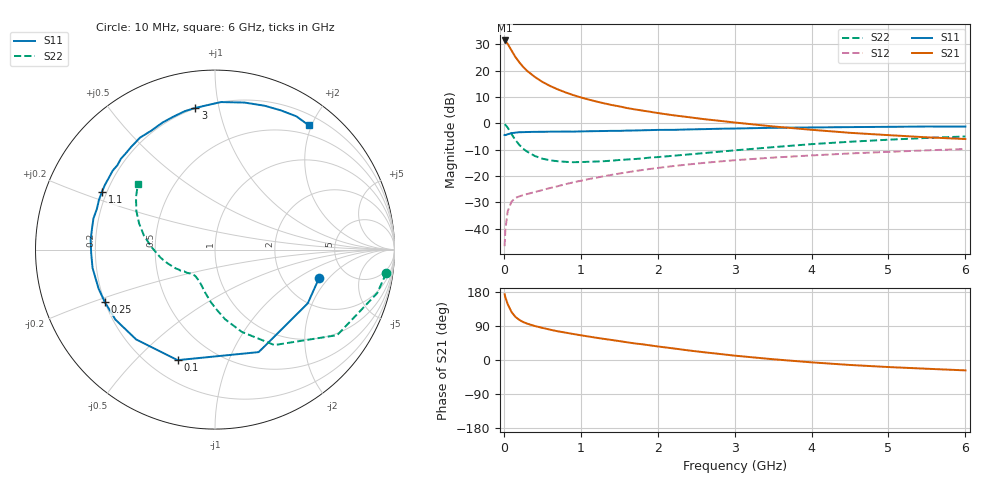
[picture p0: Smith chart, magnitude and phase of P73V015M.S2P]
! SIEMENS Small Signal Semiconductors
! BFP196
! Si NPN RF Bipolar Junction Transistor in SOT143
! VCE = 3 V  IC = 15 mA
! Common Emitter S-Parameters:  May  1996
# GHz  S  MA  R  50
!  f  S11  S21  S12  S22
! GHz  MAG  ANG  MAG  ANG  MAG  ANG  MAG  ANG
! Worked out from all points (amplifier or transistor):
!   36 points, 10 MHz to 6 GHz, reference 50 ohm
!   highest |S21| = 31.4 dB at 10 MHz (marker M1)
!   |S21| within 3 dB of that: start of sweep to 83.98 MHz
!   unconditionally stable (mu >= 1): 757.5 MHz to 3.338 GHz
!   at 250 MHz: K = 0.51, MSG = 24.3 dB, |S12| = -27.2 dB
!   at 1.4 GHz: K = 1.12, MAG = 11.1 dB, |S12| = -19.5 dB
!   at 6 GHz: K = 0.98, MSG = 1.9 dB, |S12| = -9.7 dB
!   S11 on the Smith chart (normalised r, x): 10 MHz: 3.18, -1.57; 100 MHz: 0.31, -0.67; 250 MHz: 0.20, -0.22; 1.1 GHz: 0.18, +0.23; 3 GHz: 0.20, +0.85; 6 GHz: 0.35, +1.96
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0.01  0.6013 -15.2  37.18 173.5  0.0047 84.9  0.9629 -7.8
0.02  0.5973 -30.1  35.97 165.5  0.0096 77.1  0.9358 -15.0
0.05  0.6208 -66.9  32.04 147.5  0.0215 62.9  0.8311 -35.0
0.1  0.6503 -108.7  23.99 126.6  0.0329 48.0  0.6264 -58.1
0.15  0.6661 -131.3  18.11 113.9  0.0385 40.7  0.4827 -71.9
0.2  0.6782 -144.9  14.4 106.0  0.0412 37.9  0.3927 -81.7
0.25  0.6799 -154.6  11.74 100.3  0.0436 37.0  0.3311 -88.9
0.3  0.6841 -161.4  9.954 96.2  0.0456 37.7  0.2932 -94.6
0.4  0.6899 -171.5  7.616 89.9  0.0497 39.2  0.2416 -103.8
0.5  0.6904 -178.7  6.109 84.8  0.0544 41.7  0.2138 -110.4
0.6  0.6949 175.4  5.116 80.1  0.0593 43.8  0.1993 -115.4
0.7  0.6952 170.2  4.406 75.8  0.0643 45.4  0.1911 -119.9
0.9  0.696 161.1  3.436 68.7  0.076 47.8  0.1835 -127.0
1.1  0.7075 152.9  2.827 62.0  0.0876 48.7  0.1867 -131.8
1.3  0.7145 145.5  2.399 55.7  0.0995 48.9  0.1916 -136.2
1.6  0.7287 136.0  1.949 46.8  0.1179 48.0  0.2063 -142.5
2.2  0.7517 118.2  1.423 30.7  0.1548 43.4  0.2426 -154.4
3  0.7969 97.9  1.037 11.5  0.1999 34.8  0.3075 -171.8
3.5  0.8226 87.7  0.873 2.0  0.2242 28.9  0.3534 177.8
4.5  0.8478 71.0  0.661 -13.1  0.2687 17.8  0.4478 160.9
5.5  0.87 58.6  0.543 -23.1  0.3078 6.8  0.5284 146.4
6  0.8675 53.0  0.504 -27.4  0.3261 0.9  0.5639 139.6
